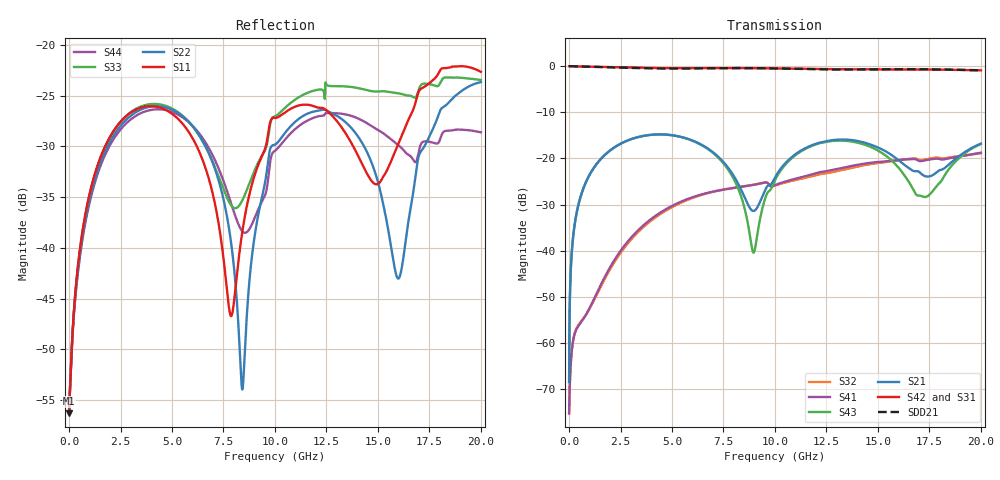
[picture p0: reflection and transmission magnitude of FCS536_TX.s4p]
!Generated from:
! 1
! 2
! 3
! 4
!PowerSI Version: 17.0.2.03131.86335  002
!Computer Host Name: W764D-PINDIS
!TouchstoneFormatFlag = 1
! GNDNET
! NETSLIST
!User Comments:
!  Touchstone file from project M5P200_FCS536_071117_85Ohm_112717
!  Exported from HFSS 3D Layout Design 2017.2.0
!  Port[1] = BGA.D30.SERDES_0_TX0_N
!  Port[2] = BGA.E30.SERDES_0_TX0_P
!  Port[3] = DIE1.410.SERDES_0_TX0_N
!  Port[4] = DIE1.411.SERDES_0_TX0_P
!  freq  S11mag  S11ang  S12mag
!  S12ang  S13mag  S13ang  S1
!  4mag  S14ang
!  S21mag  S21ang  S22mag
!  S22ang  S23mag  S23ang  S2
!  4mag  S24ang
!  S31mag  S31ang  S32mag
!  S32ang  S33mag  S33ang  S3
!  4mag  S34ang
!  S41mag  S41ang  S42mag
!  S42ang  S43mag  S43ang  S4
!  4mag  S44ang
#	Hz	S	RI	R	50
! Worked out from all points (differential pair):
!   4999 points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, 4.001 MHz to 20 GHz, reference 50 ohm
!   strongest paths, dB at 4.001 MHz, 5.001 GHz, 10 GHz, 15 GHz, 20 GHz:
!     S42: 0.0, -0.4, -0.5, -0.7, -0.9
!     S31: 0.0, -0.4, -0.5, -0.7, -0.9
!     S21: -68.4, -15.0, -24.2, -17.6, -16.8
!     S43: -68.4, -15.0, -24.7, -18.3, -16.9
!     S41: -75.2, -30.3, -25.8, -20.8, -18.8
!     S32: -75.2, -30.5, -25.9, -21.0, -18.9
!   taken as a pair (ports 2,1 in; 4,3 out), SDD21 dB: 0.0, -0.5, -0.5, -0.7, -0.9
!   lowest |S11| = -56.3 dB at 4.001 MHz (marker M1), VSWR 1.00, Z = 50.2 + j0.0139 ohm
!   |S11| at or under -10 dB: start of sweep to end of sweep
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4000800  0.00153 0.000139  0.000165 0.000342  0.9985 -0.00173  -0.000161 -6.55e-05
         0.000165 0.000342  0.00152 0.000145  -0.000161 -6.55e-05  0.9985 -0.00172
         0.9985 -0.00173  -0.000161 -6.55e-05  0.00153 0.000139  0.000165 0.000342
         -0.000161 -6.55e-05  0.9985 -0.00172  0.000165 0.000342  0.00152 0.000145
5.241048e8  0.00519 -0.00826  0.00805 0.0352  0.9721 -0.193  -0.001 -0.00127
            0.00805 0.0352  0.00547 -0.00742  -0.00105 -0.00127  0.9723 -0.1919
            0.9721 -0.193  -0.00105 -0.00127  0.00534 -0.0081  0.0085 0.0351
            -0.001 -0.00127  0.9723 -0.1919  0.0085 0.0351  0.00536 -0.00719
2.64853e9  -0.028 -0.033  0.1197 0.0899  0.5569 -0.7899  -0.00436 -0.0102
           0.1197 0.0899  -0.0242 -0.0337  -0.00417 -0.00968  0.5616 -0.7868
           0.5569 -0.7899  -0.00417 -0.00968  -0.0234 -0.0366  0.1261 0.0808
           -0.00436 -0.0102  0.5616 -0.7868  0.1261 0.0808  -0.0224 -0.0329
8.413683e9  -0.00146 -0.0119  0.0337 -0.0269  -0.9392 -0.1594  -0.0108 0.0482
            0.0337 -0.0269  -0.00173 -0.00101  -0.0107 0.0485  -0.9361 -0.1766
            -0.9392 -0.1594  -0.0107 0.0485  -0.00873 -0.0147  -0.0052 -0.035
            -0.0108 0.0482  -0.9361 -0.1766  -0.0052 -0.035  -0.0115 -0.00374
1.325065e10  -0.0378 0.00984  0.1571 0.0314  -0.0358 0.9235  0.0781 0.0117
             0.1571 0.0314  -0.0398 -0.0163  0.0741 0.0117  -0.0619 0.9219
             -0.0358 0.9235  0.0741 0.0117  -0.0351 -0.0518  0.1556 -0.00732
             0.0781 0.0117  -0.0619 0.9219  0.1556 -0.00732  -0.0371 -0.0268
1.59952e10  0.0327 0.000857  0.0924 -0.0261  0.7353 0.5559  0.058 -0.0764
            0.0924 -0.0261  0.00184 0.00682  0.0603 -0.0744  0.7156 0.5814
            0.7353 0.5559  0.0603 -0.0744  -0.0334 -0.0471  0.0194 -0.0773
            0.058 -0.0764  0.7156 0.5814  0.0194 -0.0773  -0.0283 -0.0151
2e10  -0.0277 -0.0682  0.125 0.0725  0.6472 -0.627  -0.0723 -0.0898
      0.125 0.0725  0.00365 -0.0655  -0.0748 -0.086  0.6722 -0.598
      0.6472 -0.627  -0.0748 -0.086  -0.0333 -0.0583  0.071 0.1245
      -0.0723 -0.0898  0.6722 -0.598  0.071 0.1245  -0.0255 -0.027
